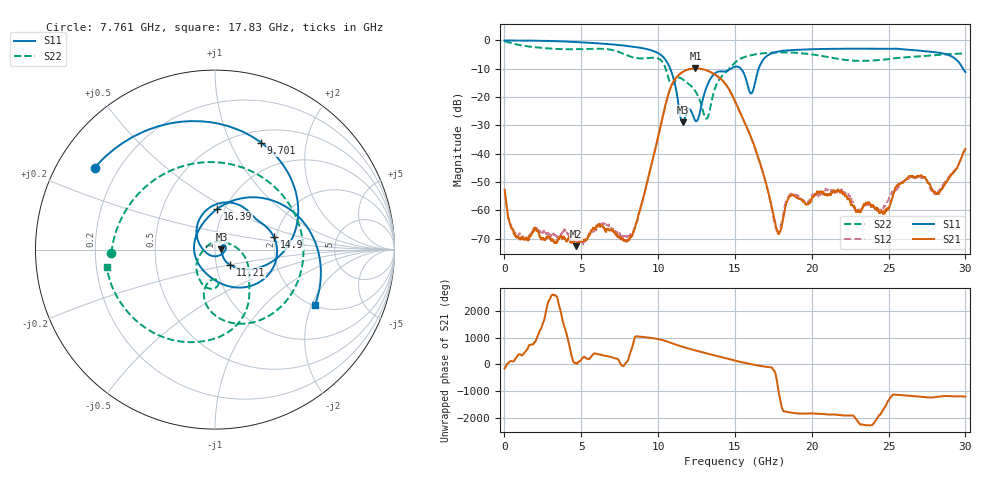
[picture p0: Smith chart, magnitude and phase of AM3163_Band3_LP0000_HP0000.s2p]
!Agilent Technologies,E8364B,MY43040894,A.07.50.67
!Agilent E8364B: A.07.50.67
!Date: Thursday, August 20, 2020 11:03:32
!Correction: S11(Full 2 Port(1,2))
!S21(Full 2 Port(1,2))
!S12(Full 2 Port(1,2))
!S22(Full 2 Port(1,2))
!S2P File: Measurements: S11, S21, S12, S22:
# Hz S  dB  R 50
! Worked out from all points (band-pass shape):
!   3201 points, 10 MHz to 30 GHz, reference 50 ohm
!   highest |S21| = -9.90 dB at 12.43 GHz (marker M1); lowest = -72.7 dB at 4.64 GHz (marker M2)
!   |S21| within 3 dB of the highest: 11.21 GHz to 13.93 GHz (2.715 GHz wide, 21.6 % of centre)
!   lowest |S11| = -28.9 dB at 11.6 GHz (marker M3), VSWR 1.07, Z = 53.7 + j0.23 ohm
!   |S11| at or under -10 dB: 10.79 GHz to 14.74 GHz (3.949 GHz wide, 30.9 % of centre); 15.39 GHz to 16.54 GHz (1.154 GHz wide, 7.23 % of centre); 29.85 GHz to end of sweep
!   |S22| runs from -27.7 to -0.4 dB; largest |S21 - S12| = 0.0046
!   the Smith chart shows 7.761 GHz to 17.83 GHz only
!   S11 on the Smith chart (normalised r, x): 7.761 GHz: 0.11, +0.30; 9.701 GHz: 0.64, +1.32; 11.21 GHz: 1.16, -0.20; 14.9 GHz: 1.95, +0.30; 16.39 GHz: 0.92, +0.44; 17.83 GHz: 2.05, -2.12
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1e7  -0.02 -1.8  -52.71 -155.3  -53.90 -175.4  -0.36 -7.4
9.284438e8  -0.05 -25.6  -69.62 14.1  -68.71 -16.8  -1.57 -85.0
2.146788e9  -0.12 -59.0  -67.11 -32.0  -66.94 56.9  -2.51 -166.6
4.639706e9  -0.57 -125.8  -72.66 61.6  -70.95 132.0  -3.13 61.0
5.014581e9  -0.69 -135.8  -71.06 -162.9  -70.09 27.5  -3.09 39.8
6.701519e9  -1.28 178.0  -66.51 -51.8  -65.18 -72.4  -3.10 -77.0
7.760541e9  -1.82 145.8  -70.56 -50.2  -68.96 75.6  -4.77 -178.1
8.622753e9  -2.41 115.6  -63.93 -33.4  -64.13 -42.5  -6.26 87.9
9.700519e9  -3.76 66.6  -41.02 -108.3  -40.99 -110.0  -6.12 -19.3
1.000979e10  -4.51 47.9  -33.86 -139.7  -34.02 -140.7  -6.42 -49.3
1.120939e10  -18.49 -45.6  -12.93 5.5  -13.01 5.5  -13.61 -87.7
1.160301e10  -28.86 3.4  -11.11 -66.7  -11.21 -66.6  -13.77 -110.1
1.242773e10  -28.40 -72.4  -9.90 158.9  -9.95 159.3  -17.98 -143.6
1.316811e10  -16.28 131.8  -10.59 48.7  -10.59 48.4  -27.63 106.5
1.490191e10  -9.47 11.7  -20.25 151.4  -20.51 151.7  -8.40 -62.9
1.5005e10  -9.26 3.8  -21.45 137.2  -21.71 137.6  -7.86 -67.3
1.639204e10  -12.87 86.7  -39.32 -31.9  -39.50 -30.6  -4.86 -123.5
1.782593e10  -3.93 -28.8  -68.26 124.1  -68.23 114.5  -4.27 -170.8
2.000958e10  -3.12 -99.8  -55.93 -26.8  -54.77 -31.8  -4.94 113.3
2.239941e10  -2.93 -155.5  -56.00 -104.5  -54.44 -116.2  -7.01 7.1
2.500479e10  -3.00 144.5  -59.30 108.1  -56.07 -28.4  -6.63 -105.5
3e10  -11.16 -20.9  -38.33 -117.6  -38.46 -116.5  -4.64 99.1
